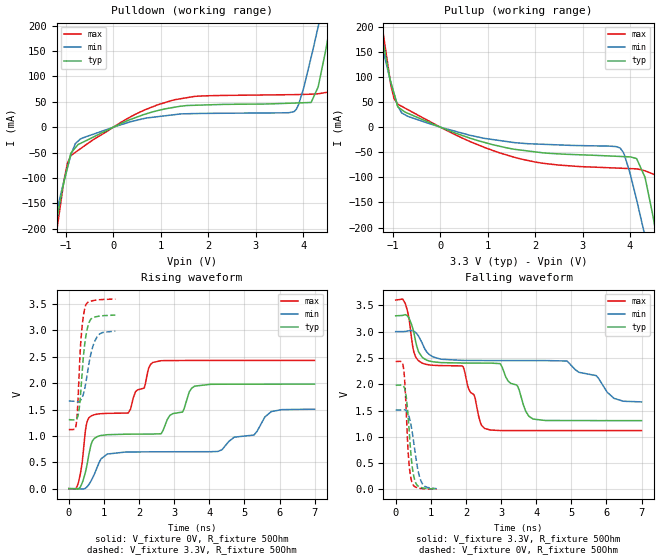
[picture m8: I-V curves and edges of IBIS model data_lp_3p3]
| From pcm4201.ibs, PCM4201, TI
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|   data_lp_3p3 Model
[Model]   data_lp_3p3
Model_type   Output
Polarity   Non-Inverting
Vmeas = 1.65
Vref = 1.65
Cref = 2pF
Rref = 50
|   typ   min   max
|   (nom PVT)   (fast PVT)   (slow PVT)
|C_comp from frequency sweep method (F=13.83MHz)
|C_comp   1.247e-12   1.127e-12   1.444e-12
|ON state : BUFFER OUTPUT TURNED HIGH
|C_comp   1.247e-12   1.127e-12   1.444e-12
|OFF state: BUFFER OUTPUT TURNED LOW
|C_comp   1.271e-12   1.187e-12   1.443e-12
|C_comp from LC tank measurement(L=1nH)
|Resonant Frequency(Hz)   7.720e+09   7.770e+09   7.500e+09
C_comp   4.254e-13   4.200e-13   4.508e-13
|ON state : BUFFER OUTPUT TURNED HIGH
|Resonant Frequency(Hz)   7.720e+09   7.770e+09   7.500e+09
|C_comp   4.254e-13   4.200e-13   4.508e-13
|OFF state: BUFFER OUTPUT TURNED LOW
|Resonant Frequency(Hz)   7.740e+09   7.900e+09   7.470e+09
|C_comp   4.232e-13   4.063e-13   4.544e-13
| Where nom  PVT is Nominal Process, 3.3V, 35C
|   Fast PVT is Strong Process,  3.6V, -10C
|   Slow PVT is Weak Process,   3V, 80C
[Voltage Range]   3.3   3   3.6
|Ambient Temperature   25   70   -10
|Junction Temperature
[Temperature Range]   35   80   -10
[Pullup Reference]   3.3   3   3.6
[Pulldown Reference]   0   0   0
[Power Clamp Reference]   3.3   3   3.6
[GND Clamp Reference]   0   0   0
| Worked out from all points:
|   slope of the pulldown table from 0 to 0.495 V, typ, clamps not added: 25 ohm
|   slope of the pullup table from 0 to 0.495 V, typ, clamps not added: 28.1 ohm
|   falling waveform, V_fixture 3.3V, R_fixture 50Ohm: 20-80 % time 3.05ns typ, 5.16ns min, 1.89ns max; typ from 3.3 V to 1.31 V
|   rising waveform, V_fixture 0V, R_fixture 50Ohm: 20-80 % time 2.81ns typ, 4.71ns min, 1.78ns max; typ from 0 V to 1.98 V
|   rising waveform, V_fixture 3.3V, R_fixture 50Ohm: 20-80 % time 163ps typ, 235ps min, 127ps max; typ from 1.31 V to 3.29 V
|   falling waveform, V_fixture 0V, R_fixture 50Ohm: 20-80 % time 148ps typ, 212ps min, 113ps max; typ from 1.98 V to 0.008 V
[Pulldown]
|   Voltage   I(typ)   I(min)   I(max)
-3.3V     -1.347A    -1.084A    -1.741A
-1.328V   -252.6mA   -221.6mA   -291.5mA
-1.104V   -136.2mA   -129.5mA   -144.6mA
-968.4mV  -79.09mA   -79.59mA   -70.65mA
-804mV    -40.75mA   -32.57mA   -49.7mA
18mV      811.1uA    603.1uA    1.128mA
1.289V    39.28mA    24.6mA     53.95mA
3.81V     47.47mA    30.76mA    64.08mA
4.316V    79.27mA    198.1mA    65.81mA
4.586V    209.9mA    313.8mA    74.95mA
4.867V    359.1mA    437.4mA    226.8mA
6.6V      1.329A     1.2A       1.496A
[Pullup]
|   Voltage   I(typ)   I(min)   I(max)
-3.3V     1.329A     1.068A     1.72A
-1.314V   224.1mA    197.1mA    257.3mA
-975.6mV  66.67mA    67.2mA     56.95mA
-693mV    27.81mA    21.83mA    35.24mA
1.559V    -44.06mA   -30.77mA   -59.99mA
3.786V    -58.33mA   -41.27mA   -81.72mA
4.138V    -62.58mA   -144.5mA   -83.06mA
4.314V    -99.37mA   -216.3mA   -86.96mA
4.511V    -191.4mA   -299.6mA   -94.31mA
4.59V     -233.5mA   -333.5mA   -102.1mA
4.871V    -382.5mA   -456.2mA   -254.8mA
6.6V      -1.347A    -1.218A    -1.518A
[Ramp]
R_load = 50
|   typ   min   max
dV/dt_r   1.18901/2.81103e-09   0.903979/4.70574e-09   1.45875/1.78614e-09
dV/dt_f   1.19482/3.05129e-09   0.801605/5.15319e-09   1.48886/1.88926e-09
[Falling Waveform]
V_fixture = 3.3V
V_fixture_min = 3V
V_fixture_max = 3.6V
R_fixture = 50Ohm
|   Time   V(typ)   V(min)   V(max)
0s        3.3V       3V         3.6V
269ps     3.321V     3.003V     3.543V
644ps     2.629V     2.921V     2.451V
1.07ns    2.425V     2.518V     2.36V
1.916ns   2.403V     2.453V     2.338V
2.528ns   2.402V     2.451V     1.161V
2.978ns   2.388V     2.45V      1.12V
3.914ns   1.338V     2.45V      1.119V
4.874ns   1.31V      2.441V     1.118V
6.998ns   1.308V     1.664V     1.118V
[Rising Waveform]
V_fixture = 0V
V_fixture_min = 0V
V_fixture_max = 0V
R_fixture = 50Ohm
|   Time   V(typ)   V(min)   V(max)
0s        117uV      80.69uV    163.6uV
269ps     -8.106mV   -792.2uV   105.2mV
566ps     626.9mV    73.34mV    1.337V
920ps     1.009V     566.4mV    1.422V
1.691ns   1.033V     694mV      1.435V
2.393ns   1.035V     698mV      2.393V
3.584ns   1.944V     699.9mV    2.431V
5.27ns    1.981V     1.016V     2.431V
5.768ns   1.982V     1.462V     2.431V
6.998ns   1.982V     1.507V     2.431V
[Rising Waveform]
V_fixture = 3.3V
V_fixture_min = 3V
V_fixture_max = 3.6V
R_fixture = 50Ohm
|   Time   V(typ)   V(min)   V(max)
0s        1.309V     1.661V     1.119V
215ps     1.318V     1.65V      1.237V
245ps     1.349V     1.648V     1.476V
296ps     1.519V     1.656V     2.213V
344ps     1.872V     1.686V     2.813V
413ps     2.488V     1.79V      3.265V
479ps     2.864V     1.987V     3.474V
596ps     3.18V      2.455V     3.55V
809ps     3.266V     2.884V     3.579V
1.325ns   3.293V     2.987V     3.596V
[Falling Waveform]
V_fixture = 0V
V_fixture_min = 0V
V_fixture_max = 0V
R_fixture = 50Ohm
|   Time   V(typ)   V(min)   V(max)
0s        1.982V     1.508V     2.431V
167ps     1.987V     1.512V     2.428V
224ps     1.963V     1.515V     2.304V
257ps     1.914V     1.512V     2.057V
296ps     1.783V     1.496V     1.555V
368ps     1.262V     1.41V      585.4mV
464ps     468.2mV    1.118V     133.8mV
560ps     141.1mV    671.3mV    47.16mV
713ps     38.8mV     172.8mV    19.11mV
1.169ns   8.178mV    14.03mV    5.627mV
